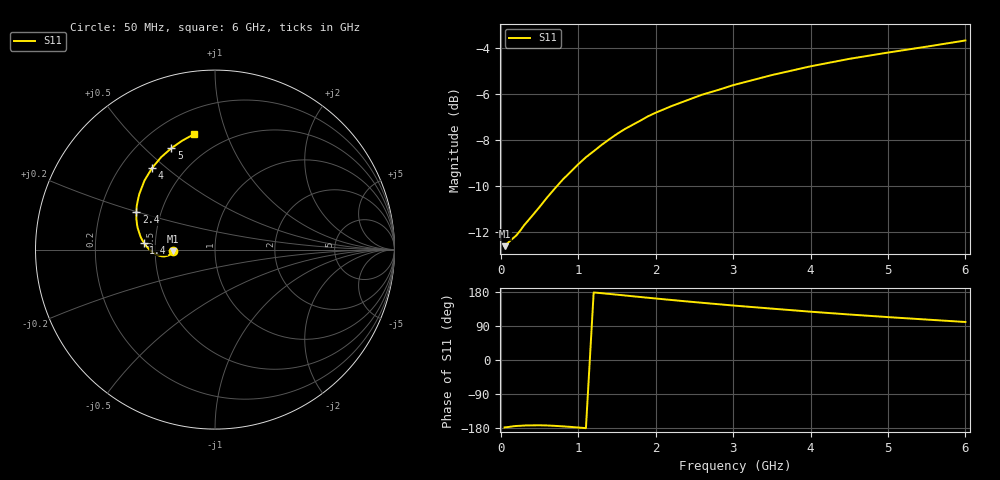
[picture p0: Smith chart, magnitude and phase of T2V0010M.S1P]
! SIEMENS Discrete & RF Semiconductors
! BAS70-04W
! Si Schottky Diode in SOT323
! IF = 10 mA
! S-Parameters:  November  1997
# GHz  S  MA  R  50
!  f  S11
! GHz  MAG  ANG
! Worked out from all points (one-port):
!   34 points, 50 MHz to 6 GHz, reference 50 ohm
!   lowest |S11| = -12.6 dB at 50 MHz (marker M1), VSWR 1.61, Z = 31 - j0.537 ohm
!   |S11| at or under -10 dB: start of sweep to 727.1 MHz
!   S11 on the Smith chart (normalised r, x): 50 MHz: 0.62, -0.01; 1.4 GHz: 0.43, +0.04; 2.4 GHz: 0.36, +0.20; 4 GHz: 0.33, +0.45; 5 GHz: 0.33, +0.61; 6 GHz: 0.34, +0.77
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0.05  0.2343 -178.0
0.1  0.2388 -176.8
0.15  0.243 -175.2
0.2  0.247 -174.1
0.3  0.2598 -172.9
0.5  0.2847 -172.3
0.6  0.2988 -172.8
0.7  0.3125 -173.8
0.8  0.3264 -175.1
0.9  0.3391 -176.5
1  0.3524 -178.1
1.1  0.365 -179.9
1.3  0.388 176.4
1.4  0.399 174.4
1.5  0.4099 172.4
1.6  0.42 170.4
1.9  0.4476 164.3
2  0.4558 162.3
2.2  0.4708 158.5
2.4  0.4846 154.6
2.6  0.4988 151.0
3  0.523 143.8
3.5  0.55 135.6
4  0.5746 127.5
4.5  0.5964 120.1
5  0.6154 113.2
5.5  0.6339 106.7
6  0.6537 100.3
